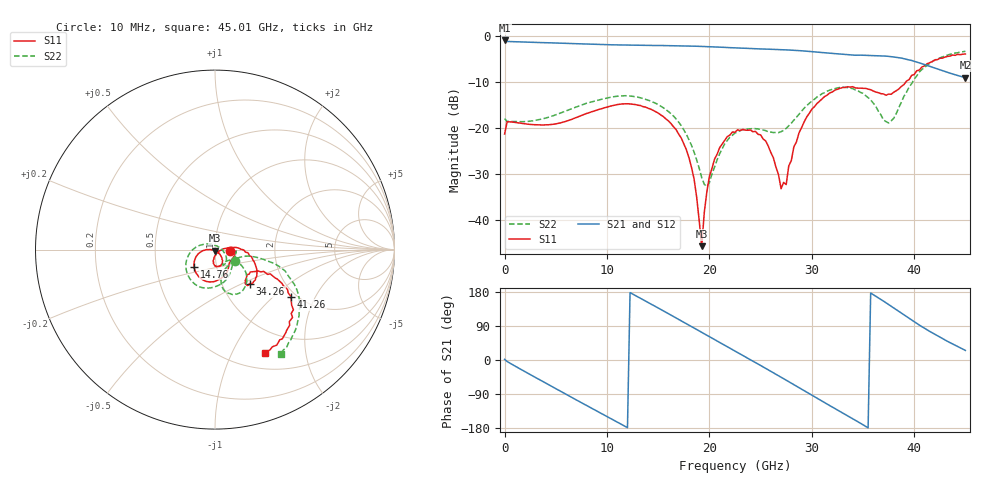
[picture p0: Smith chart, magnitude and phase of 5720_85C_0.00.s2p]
! Device:  ADRF5720
! Description: 0.5dB LSB GaAs MMIC 6-bit Digital Attenuator
! Frequency:  0.000009 -  40 GHz
! Ports:
!	RF1	= Port 1
!	RF2	= Port 2
! Vdd:  3.3 Volt
! Vss:  -3.3 Volt
! Control:  0/3.3 Volt
! State:  0.00 dB attenuation
! Data:  The device was measured using G-S-G Probes on a matrix board.
!  Data was collected using an calibrated 4 port network analyzer.
!  The reference plane for this measurement is at the launchers.
! Note:  Analog Devices supplies this data as a sample of measured data
!  for this product.  Your particular data for this product may vary.
!  Data was taken at 85 degrees C.
!  Analog Devices reserves the right to change this data at anytime.
# GHZ S DB R 45.0
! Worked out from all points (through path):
!   181 points, 10 MHz to 45.01 GHz, reference 45 ohm
!   highest |S21| = -0.93 dB at 10 MHz (marker M1); lowest = -9.0 dB at 45.01 GHz (marker M2)
!   group delay of S21, straight-line fit = 42.9 ps
!   lowest |S11| = -45.8 dB at 19.26 GHz (marker M3), VSWR 1.01, Z = 45.1 - j0.458 ohm
!   |S11| at or under -10 dB: start of sweep to 39.19 GHz
!   |S22| runs from -32.8 to -3.3 dB; largest |S21 - S12| = 0.0044
!   S11 on the Smith chart (normalised r, x): 10 MHz: 1.19, -0.02; 14.76 GHz: 0.78, -0.15; 34.26 GHz: 1.35, -0.56; 41.26 GHz: 1.87, -1.32; 45.01 GHz: 0.69, -1.35
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0.01  -21.32 -6.7  -0.93 1.8  -0.92 1.8  -17.95 -30.8
0.26  -18.63 -4.3  -1.15 -4.1  -1.14 -4.0  -18.57 -3.9
4.01  -19.31 -38.8  -1.42 -60.8  -1.40 -60.7  -17.84 -39.7
7.76  -17.08 -60.8  -1.69 -116.3  -1.67 -116.2  -14.81 -71.4
11.26  -14.83 -96.7  -1.92 -167.6  -1.90 -167.4  -13.03 -107.9
14.76  -16.46 -140.8  -2.02 140.9  -2.01 141.1  -14.62 -151.0
15.26  -17.16 -147.1  -2.04 133.5  -2.02 133.6  -15.24 -157.6
18.01  -26.44 179.5  -2.14 92.0  -2.12 92.2  -22.54 158.0
18.51  -31.06 178.6  -2.17 84.4  -2.15 84.5  -25.23 144.2
19.26  -45.75 -80.3  -2.23 72.9  -2.21 73.1  -30.82 108.2
19.76  -33.93 -40.3  -2.27 65.3  -2.25 65.5  -32.77 58.5
20.51  -26.80 -46.2  -2.34 53.8  -2.32 54.0  -28.55 1.0
22.76  -20.40 -70.2  -2.57 19.7  -2.55 19.9  -20.86 -46.7
25.51  -22.84 -95.8  -2.81 -22.1  -2.79 -21.9  -20.58 -62.6
27.01  -33.23 -68.6  -2.94 -45.4  -2.92 -45.2  -20.81 -43.5
27.51  -32.33 -15.6  -2.99 -53.2  -2.97 -53.0  -20.08 -36.4
28.76  -21.07 8.3  -3.15 -73.0  -3.13 -72.8  -16.99 -29.6
30.26  -15.38 -4.8  -3.42 -96.8  -3.40 -96.6  -13.76 -35.1
34.26  -11.26 -44.5  -4.15 -159.0  -4.13 -158.7  -11.72 -70.9
37.76  -12.65 -32.3  -4.46 141.9  -4.44 142.2  -18.45 -33.7
41.26  -6.02 -31.9  -6.37 79.7  -6.35 80.1  -6.34 -23.6
45.01  -3.88 -64.2  -9.01 25.3  -8.98 25.7  -3.29 -57.7
